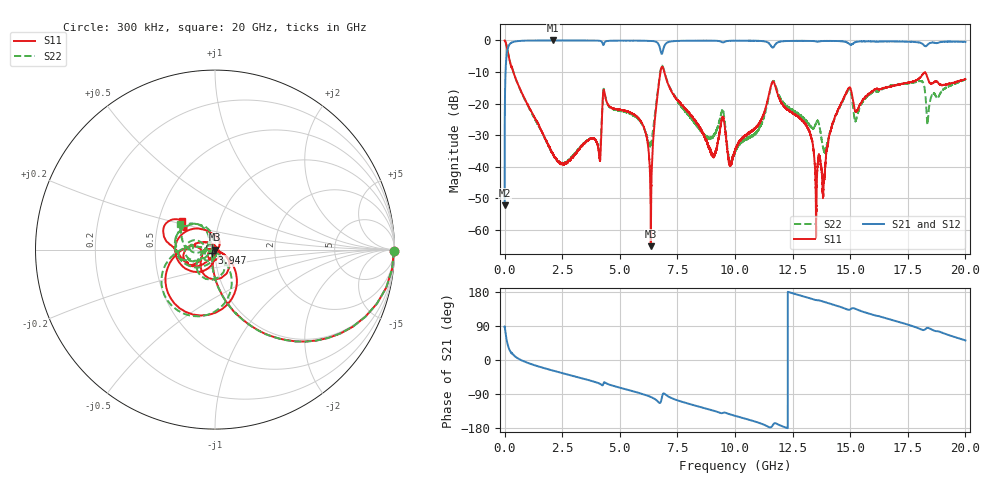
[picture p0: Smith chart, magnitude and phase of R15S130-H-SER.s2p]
!{R15S130}
!Johanson Technology Inc.
!www.johansontechnology.com
!Test Board Conditions:
!Substrate Type  RO4350B
!Substrate Thickness  20 mil
!Substrate Dk  3.66
!TL Type: GCPW
!TL Trace Width  34 mil
!TL Gap  10 mil
!Electrode orientation  Horizontal
!DUT TOPOLOGY	SERIES
!Mounting Pad LxW  26x52 mil
! Created Sat Feb  6 14:10:44 2021
# hz S ma R 50
! 2 Port Network Data from SP1.SP block
! freq  magS11  angS11  magS21  angS21  magS12  angS12  magS22  angS22
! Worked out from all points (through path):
!   20001 points, 300 kHz to 20 GHz, reference 50 ohm
!   highest |S21| = 0.00 dB at 2.111 GHz (marker M1); lowest = -52.2 dB at 300 kHz (marker M2)
!   group delay of S21, straight-line fit = 43.5 ps
!   lowest |S11| = -65.2 dB at 6.345 GHz (marker M3), VSWR 1.00, Z = 50 - j0.0282 ohm
!   |S11| at or under -10 dB: 380.3 MHz to 6.763 GHz (6.382 GHz wide, 179 % of centre); 6.932 GHz to end of sweep
!   |S22| runs from -39.5 to 0.0 dB; largest |S21 - S12| = 0.014
!   S11 on the Smith chart (normalised r, x): 300 kHz: open; 3.947 GHz: 0.96, -0.04; 20 GHz: 0.66, +0.22
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300000  0.9971 -0.3  0.002465 87.8  0.002496 89.3  0.9968 -0.3
1.043e8  0.7576 -42.0  0.6489 47.8  0.6503 47.8  0.7579 -42.0
2.053e8  0.5063 -62.1  0.8591 27.6  0.8588 27.6  0.5068 -62.1
2.1113e9  0.01558 -107.4  0.9998 -28.2  0.9983 -28.2  0.01552 -126.2
3.3343e9  0.02099 -119.5  0.9975 -48.0  0.9978 -48.0  0.02156 -145.3
3.9473e9  0.02647 -133.7  0.995 -58.4  0.9955 -58.4  0.02639 -146.1
4.1183e9  0.01365 -106.2  0.9878 -62.2  0.9882 -62.3  0.01646 -109.8
4.3563e9  0.1363 -123.7  0.9466 -59.4  0.9457 -59.5  0.1377 -138.4
5.9303e9  0.05109 178.1  0.991 -88.7  0.9924 -88.7  0.04934 -168.1
6.3453e9  0.0005514 -149.3  0.9844 -97.4  0.9852 -97.4  0.02217 -97.3
6.6673e9  0.1682 -47.0  0.8909 -110.4  0.8892 -110.3  0.1798 -59.5
9.0333e9  0.01538 50.6  0.9899 -133.1  0.9915 -133.2  0.03005 -123.5
9.4523e9  0.06032 -97.5  0.9334 -140.0  0.9351 -140.1  0.07984 -135.0
1.00003e10  0.01791 -84.3  0.9901 -147.3  0.9901 -147.3  0.01734 -80.5
1.16483e10  0.2219 -177.5  0.7705 -171.2  0.7722 -171.2  0.2268 171.2
1.33343e10  0.02694 33.9  0.9812 161.4  0.9823 161.2  0.04128 118.6
1.38323e10  0.004138 -25.5  0.9796 154.1  0.9814 154.1  0.01973 136.9
1.49003e10  0.1692 -149.8  0.9152 132.9  0.9138 132.7  0.161 -165.5
1.52513e10  0.07529 -166.9  0.9466 134.6  0.949 134.7  0.05493 -167.4
1.66673e10  0.1832 -161.3  0.9679 108.2  0.9571 108.2  0.1875 -162.0
1.83823e10  0.2402 139.5  0.8723 84.7  0.8722 84.8  0.05954 -178.9
2e10  0.2441 138.9  0.9484 51.7  0.9417 51.4  0.2423 143.6
